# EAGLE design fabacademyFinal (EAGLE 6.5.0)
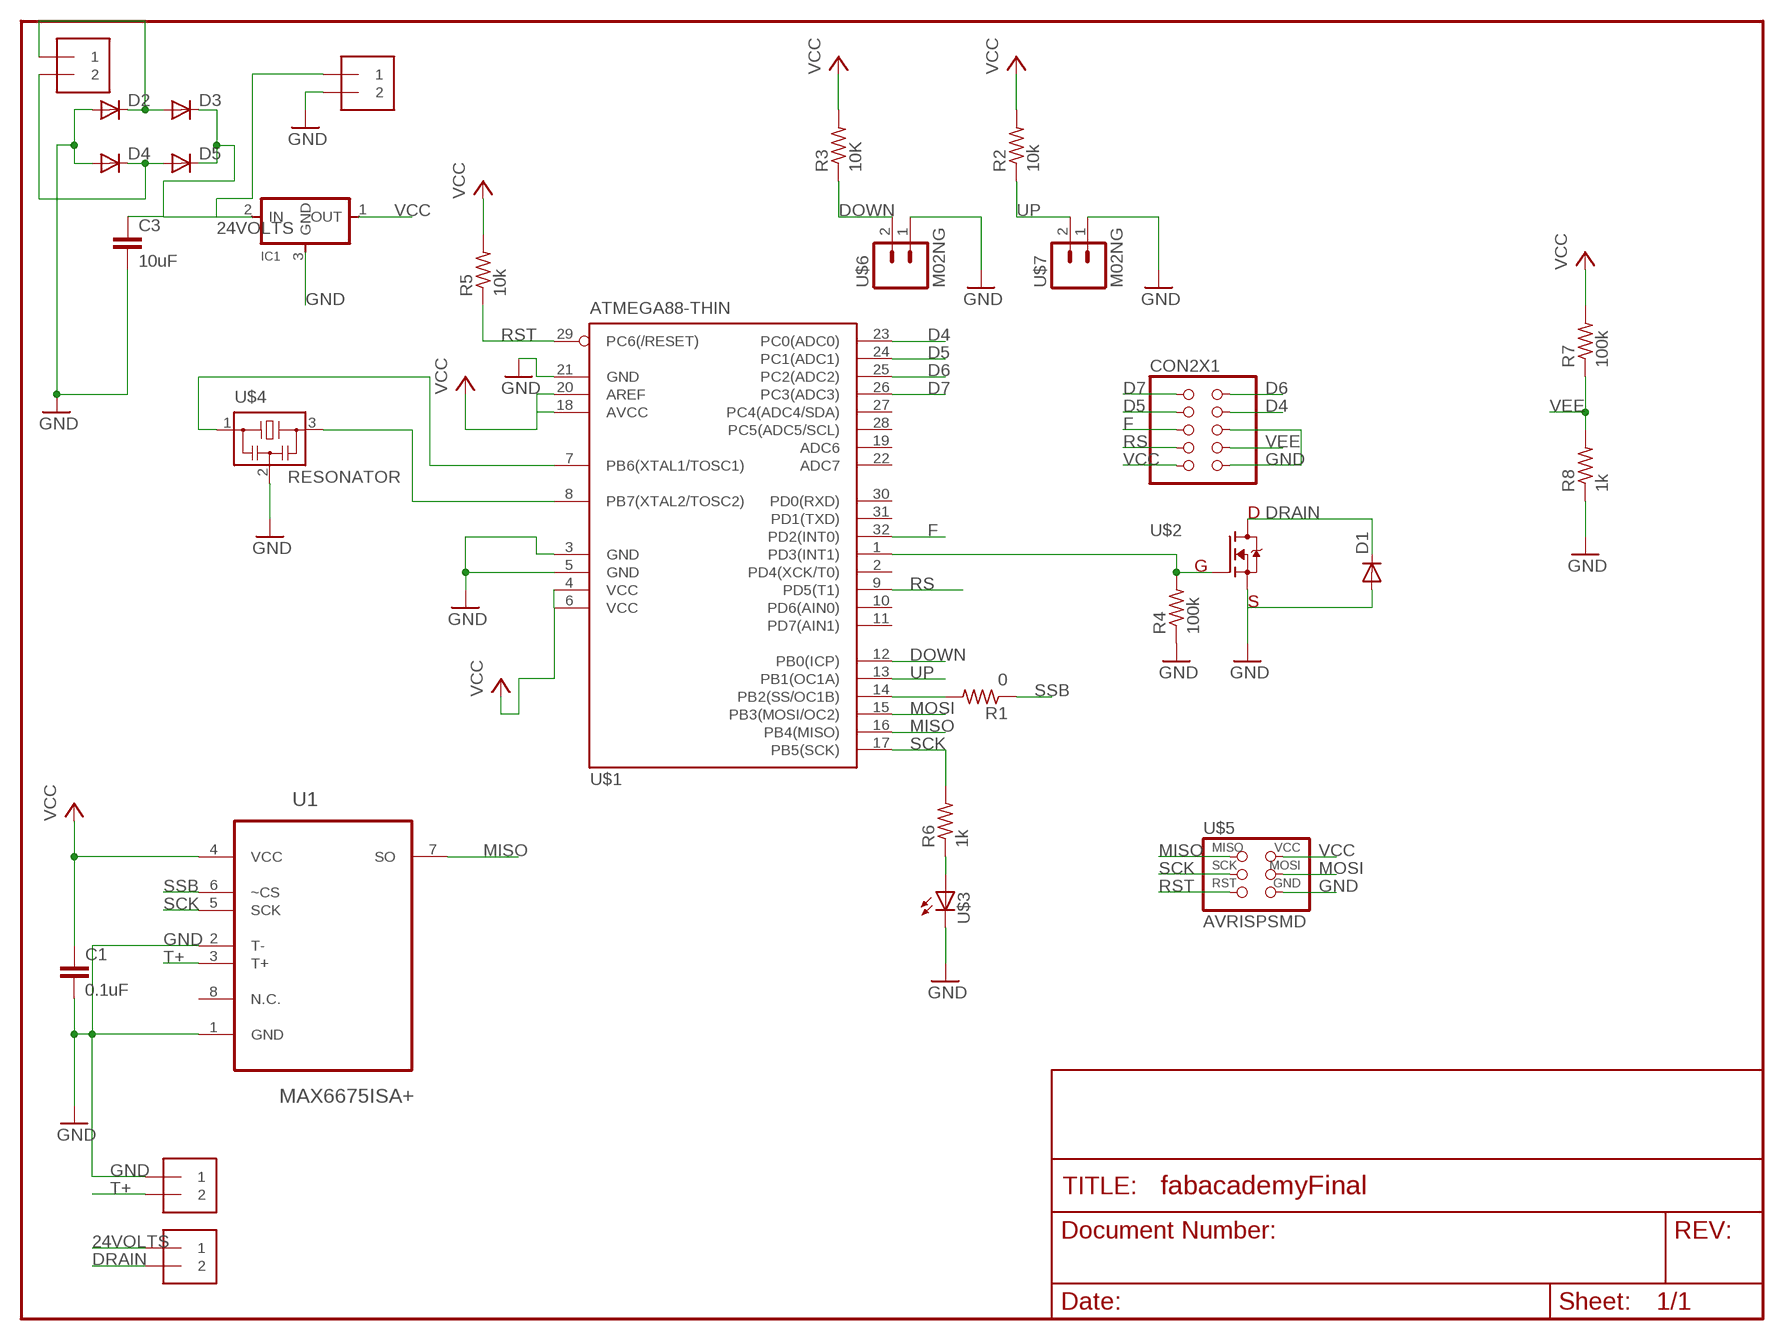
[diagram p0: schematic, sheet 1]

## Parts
C1  0.1uF  CAP1206  [1206]
C3  10uF  CAP1206  [1206]
CON2X1  CONN2X05  [2X05SMD]
D1  DIODESOD123  [SOD123]
D2  DIODESOD123  [SOD123]
D3  DIODESOD123  [SOD123]
D4  DIODESOD123  [SOD123]
D5  DIODESOD123  [SOD123]
IC1  REGULATORSOT23  [SOT23]
J1  1X2-3.5MM  [3.5MMTERM]
J2  1X2-3.5MM  [3.5MMTERM]
J3  1X2-3.5MM  [3.5MMTERM]
J4  1X2-3.5MM  [3.5MMTERM]
R1  0  RESISTOR1206  [1206]
R2  10k  RESISTOR1206  [1206]
R3  10K  RESISTOR1206  [1206]
R4  100k  RESISTOR1206  [1206]
R5  10k  RESISTOR1206  [1206]
R6  1k  RESISTOR1206  [1206]
R7  100k  RESISTOR1206  [1206]
R8  1k  RESISTOR1206  [1206]
U1  MAX6675ISA+  [SOIC127P600X175-8N]
U$1  ATMEGA88-THIN  [TQFP32-08THIN]
U$2  N-MOSFETTO-252  [N-MOSFET]
U$3  LED1206  [1206]
U$4  RESONATOR  [EFOBM]
U$5  AVRISPSMD  [2X03SMD]
U$6  M02NG  [1X02]
U$7  M02NG  [1X02]

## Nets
24VOLTS: C3.1 D3.CATHODE(C) D5.CATHODE(C) IC1.2(IN) J1.1 J2.1
D4: CON2X1.7(DB4) U$1.23(PC0(ADC0))
D5: CON2X1.8(DB5) U$1.24(PC1(ADC1))
D6: CON2X1.9(DB6) U$1.25(PC2(ADC2))
D7: CON2X1.10(DB7) U$1.26(PC3(ADC3))
DOWN: R3.1 U$1.12(PB0(ICP)) U$6.2
DRAIN: D1.CATHODE(C) J2.2 U$2.3(D)
F: CON2X1.6(E) U$1.32(PD2(INT0))
GND: C1.2 C3.2 CON2X1.1(GND) CON2X1.5(R/W) D1.ANODE(A) D2.ANODE(A) D4.ANODE(A) IC1.3(GND) J1.2 J3.1 R4.1 R8.1 U1.1(GND) U1.2(T-) U$1.3(GND) U$1.5(GND) U$1.21(GND) U$2.2(S) U$3.2(C) U$4.2 U$5.6(GND) U$6.1 U$7.1
MISO: U1.7(SO) U$1.16(PB4(MISO)) U$5.1(MISO)
MOSI: U$1.15(PB3(MOSI/OC2)) U$5.4(MOSI)
N$1: D2.CATHODE(C) D3.ANODE(A) J4.1
N$2: D4.CATHODE(C) D5.ANODE(A) J4.2
N$3: R4.2 U$1.1(PD3(INT1)) U$2.1(G)
N$4: U$1.8(PB7(XTAL2/TOSC2)) U$4.3
N$5: U$1.7(PB6(XTAL1/TOSC1)) U$4.1
N$6: R6.1 U$3.1(A)
N$7: R1.2 U$1.14(PB2(SS/OC1B))
RS: CON2X1.4(RS) U$1.9(PD5(T1))
RST: R5.1 U$1.29(PC6(/RESET)) U$5.5(RST)
SCK: R6.2 U1.5(SCK) U$1.17(PB5(SCK)) U$5.3(SCK)
SSB: R1.1 U1.6(~CS)
T+: J3.2 U1.3(T+)
UP: R2.1 U$1.13(PB1(OC1A)) U$7.2
VCC: C1.1 CON2X1.2(VCC) IC1.1(OUT) R2.2 R3.2 R5.2 R7.2 U1.4(VCC) U$1.4(VCC) U$1.6(VCC) U$1.18(AVCC) U$1.20(AREF) U$5.2(VCC)
VEE: CON2X1.3(VEE) R7.1 R8.2
Unconnected: U1.8(N.C.) U$1.2(PD4(XCK/T0)) U$1.10(PD6(AIN0)) U$1.11(PD7(AIN1)) U$1.19(ADC6) U$1.22(ADC7) U$1.27(PC4(ADC4/SDA)) U$1.28(PC5(ADC5/SCL)) U$1.30(PD0(RXD)) U$1.31(PD1(TXD))

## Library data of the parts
C1 C3 = 01_SparkFun:CAP: Capacitor
CON2X1 = 01_ng:CONN2X05
D1-D5 = 01_ng:DIODE: DIODE
IC1 = 01_ng:REGULATOR
J1-J4 = 01_adafruit:1X2: 3.5mm Terminal block
R1-R8 = 01_ng:RESISTOR
U1 = Maxim_By_element14_Batch_1:MAX6675ISA+: Cold-Junction-Compensated K-Thermocoupleto-to-; MPN: MAX6675ISA+; OC_FARNELL: 1379740; OC_NEWARK: 68K4982; PACKAGE: SOIC-8; SUPPLIER: Maxim
U$1 = 01_fab:ATMEGA88-THIN
U$2 = 01_Ali:N-MOSFET
U$3 = 01_ng:LED
U$4 = 01_fab:RESONATOR
U$5 = 01_FAB_Hello:AVRISP
U$6 U$7 = 01_SparkFun:M02NG

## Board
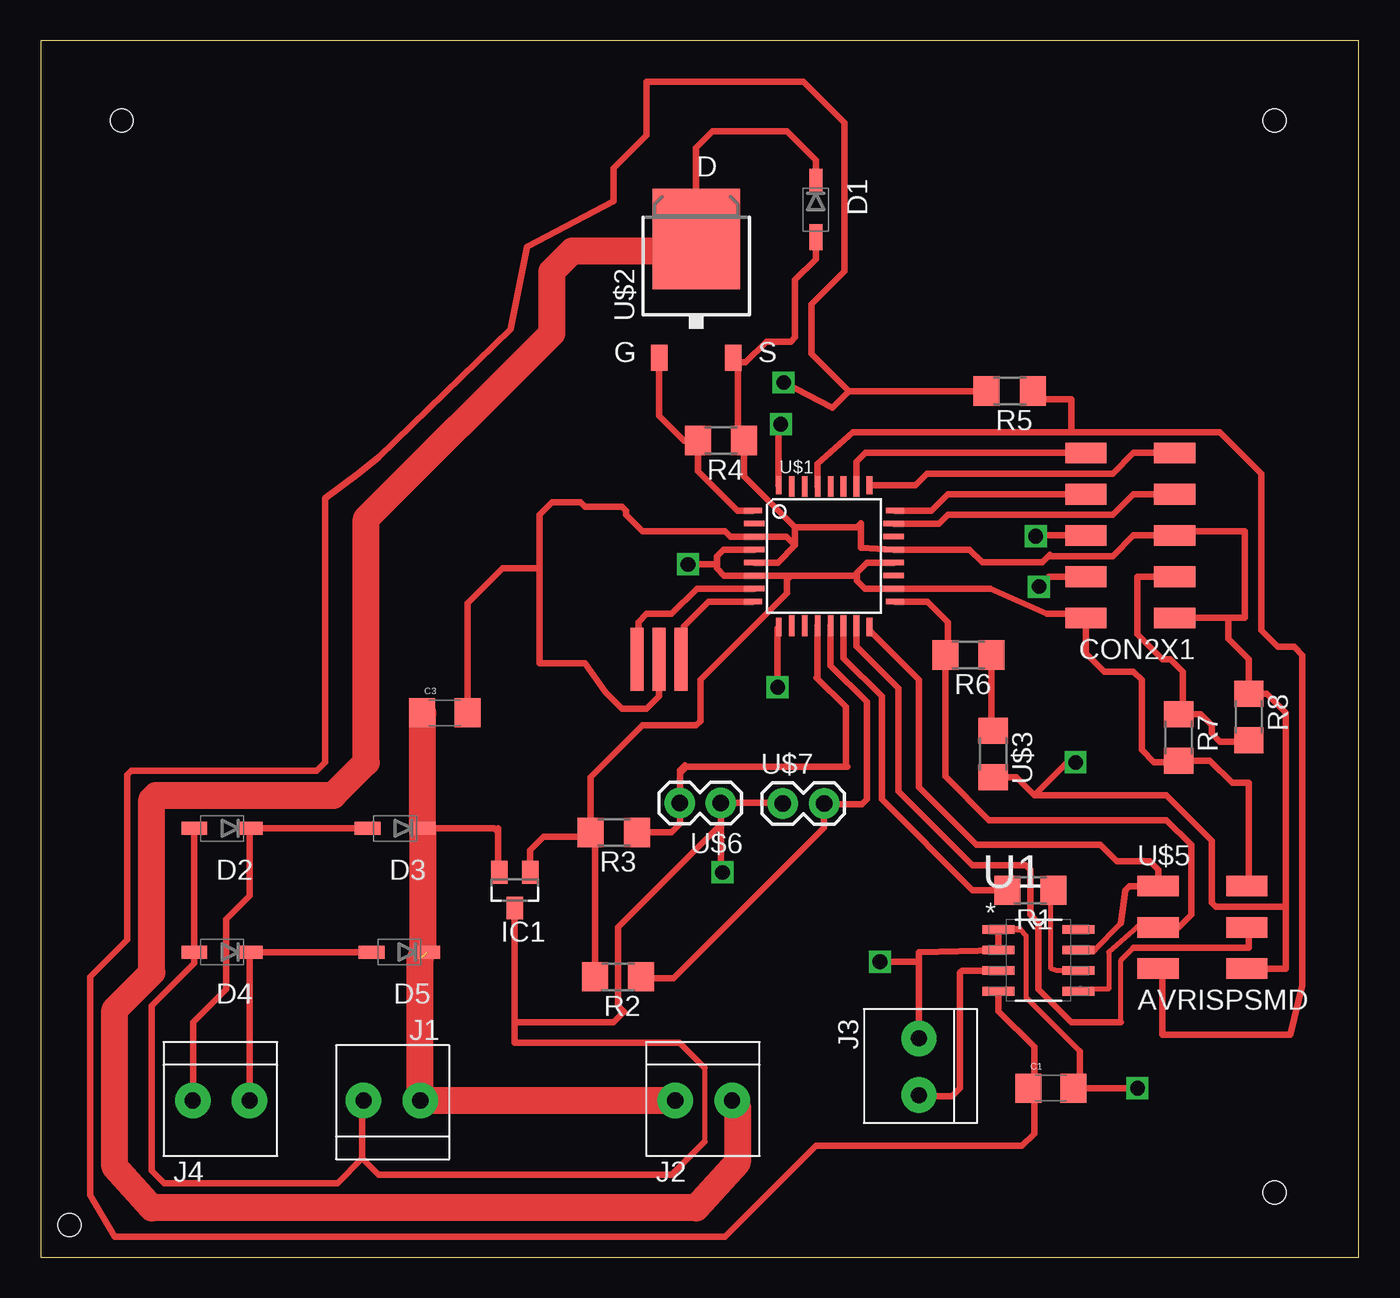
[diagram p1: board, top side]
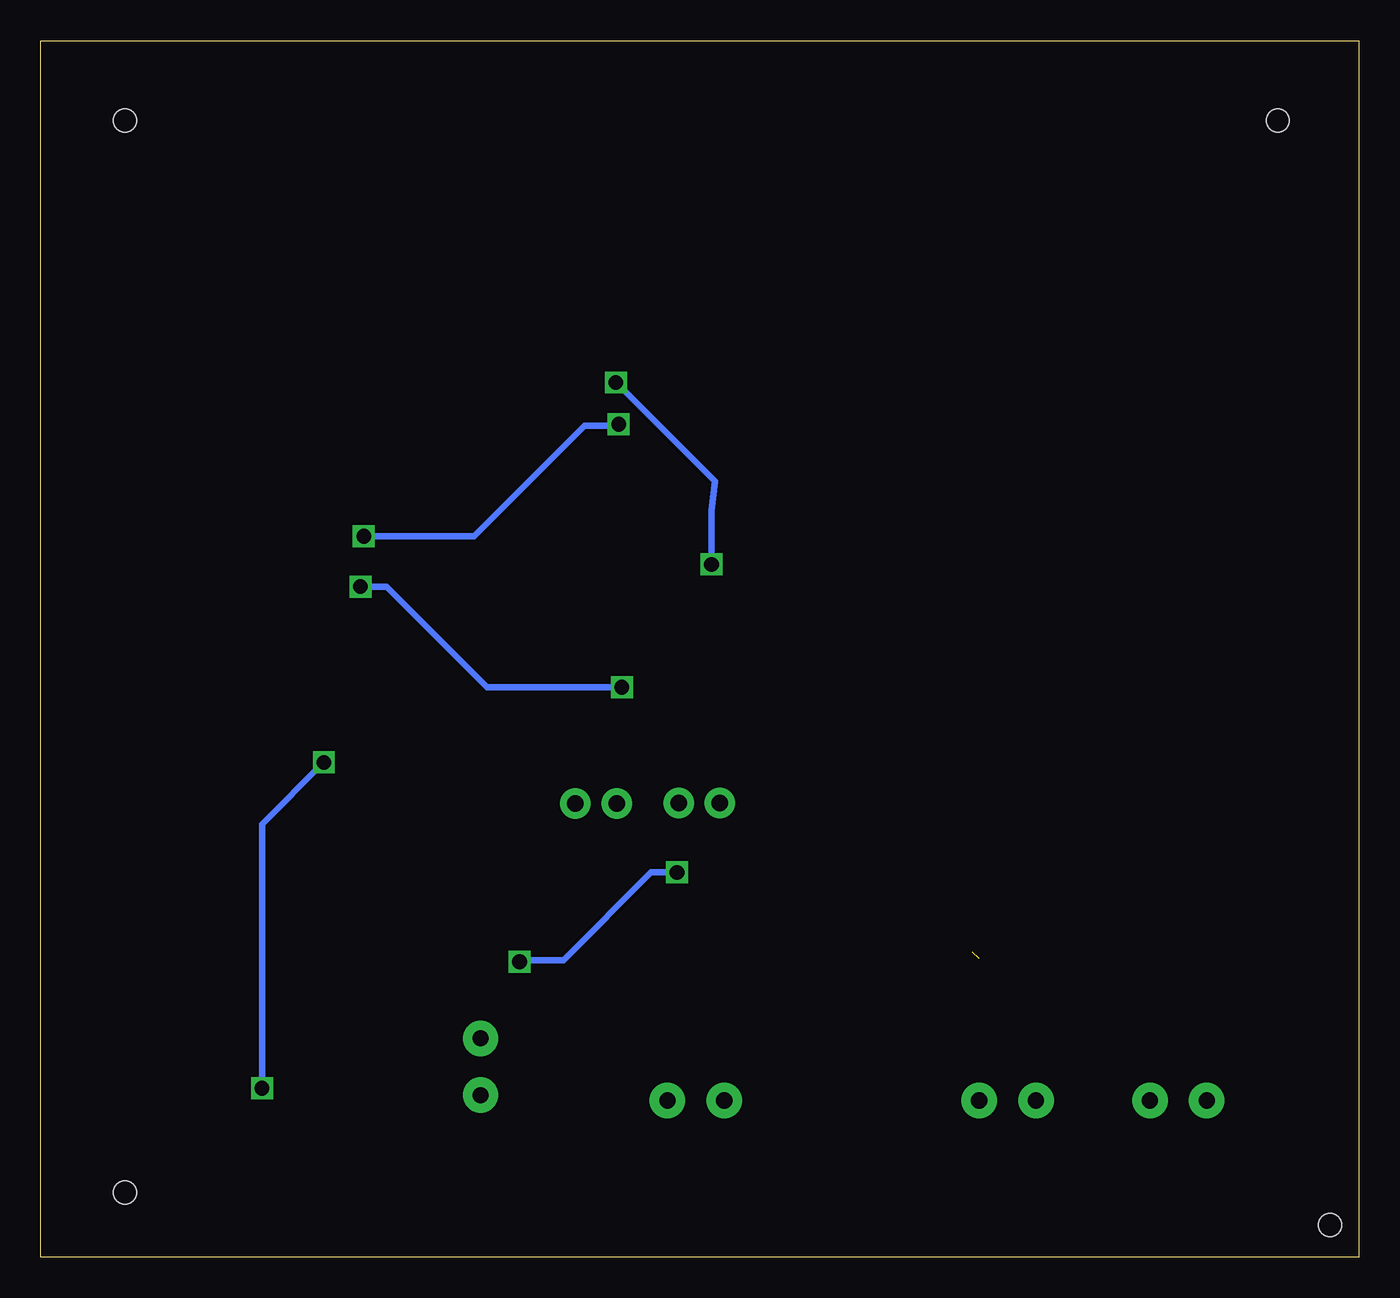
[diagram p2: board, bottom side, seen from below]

Size 81.2 x 74.92 mm. Coordinates in mm from the lower left corner, seen from the top.
Outline: 0,0 81.2,0 81.2,74.92 0,74.92 0,0
Copper layers (1*16): Top 0.035mm / dielectric 1.5mm / Bottom 0.035mm
Design rules "default *": minimum track width 16mil, minimum drill 24mil, track to track 15mil, track to pad 15mil, pad to pad 16mil, via to via 16mil, smd to smd 8mil, copper to edge 40mil, drill to drill 8mil, minimum pad ring 10mil, minimum via ring 8mil, stop-mask expansion 4mil, vias tented up to drill 0mil, thermal gap 10mil
Holes 1.4 mm at 76,70 5,70 76,4 1.78,2

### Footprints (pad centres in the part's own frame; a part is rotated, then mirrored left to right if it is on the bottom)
1206 = smd 1.6 x 1.8: 1 -1.4,0; 2 1.4,0
2X05SMD = smd 2.54 x 1.27: 1 -2.54,3.81; 2 2.92,3.81; 3 -2.54,1.27; 4 2.92,1.27; 5 -2.54,-1.27; 6 2.92,-1.27; 7 -2.54,-3.81; 8 2.92,-3.81; 9 -2.54,-6.35; 10 2.92,-6.35
SOD123 = smd 1.6 x 0.8: ANODE 1.7,0; CATHODE -1.7,0
SOT23 = smd 1 x 1.4: 1 -0.95,-1.1; 2 0.95,-1.1; 3 0,1.1
3.5MMTERM = drill 1 pad 2.184: 1 1.8,0; 2 -1.7,0
1206' = smd 1.6 x 1.803: 1 -1.422,0; 2 1.422,0
SOIC127P600X175-8N = smd 1.981 x 0.533: 1 -2.464,1.905; 2 -2.464,0.635; 3 -2.464,-0.635; 4 -2.464,-1.905; 5 2.464,-1.905; 6 2.464,-0.635; 7 2.464,0.635; 8 2.464,1.905
TQFP32-08THIN = smd 1.118 x 0.356: 1 -4.369,2.8; 8 -4.369,-2.8; 17 4.369,-2.8; 24 4.369,2.8 | smd 1.27 x 0.356: 2 -4.293,2; 3 -4.293,1.2; 4 -4.293,0.4; 5 -4.293,-0.4; 6 -4.293,-1.2; 7 -4.293,-2; 18 4.293,-2; 19 4.293,-1.2; 20 4.293,-0.4; 21 4.293,0.4; 22 4.293,1.2; 23 4.293,2 | smd 0.356 x 1.118: 9 -2.8,-4.369; 16 2.8,-4.369; 25 2.8,4.369; 32 -2.8,4.369 | smd 0.356 x 1.27: 10 -2,-4.293; 14 1.2,-4.293; 15 2,-4.293; 26 2,4.293; 27 1.2,4.293; 31 -2,4.293 | smd 0.35 x 1.27: 11 -1.2,-4.293; 12 -0.4,-4.293; 13 0.4,-4.293; 28 0.4,4.293; 29 -0.4,4.293; 30 -1.2,4.293
N-MOSFET = smd 1 x 1.6: 1 -2.28,-4.8; 2 2.28,-4.8 | smd 5.4 x 6.2: 3 0,2.5
EFOBM = smd 0.8 x 3.9: 1 -1.35,0; 2 0,0; 3 1.35,0
2X03SMD = smd 2.54 x 1.27: 1 -2.54,2.54; 2 2.92,2.54; 3 -2.54,0; 4 2.92,0; 5 -2.54,-2.54; 6 2.92,-2.54
1X02 = drill 1.016 pad 1.88: 1 0,0; 2 2.54,0

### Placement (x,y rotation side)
C1  62.23,10.41 0 top
C3  24.89,33.53 0 top
CON2X1  67.31,43.18 180 top
D1  47.75,64.52 270 top
D2  11.18,26.42 180 top
D3  21.84,26.42 180 top
D4  11.18,18.8 180 top
D5  22.1,18.8 180 top
IC1  29.21,22.61 180 top
J1  21.59,9.65 0 top
J2  40.89,9.65 180 top
J3  54.1,11.68 90 top
J4  11.18,9.65 180 top
R1  0  [1206']  60.96,22.61 180 top
R2  10k  [1206']  35.56,17.27 180 top
R3  10K  [1206']  35.31,26.16 180 top
R4  100k  [1206']  41.91,50.29 180 top
R5  10k  [1206']  59.69,53.34 180 top
R6  1k  [1206']  57.15,37.08 180 top
R7  100k  [1206']  70.1,32 270 top
R8  1k  [1206']  74.42,33.27 270 top
U1  61.47,18.29 0 top
U$1  48.26,43.18 0 top
U$2  40.39,60.2 0 top
U$3  [1206']  58.67,30.99 270 top
U$4  38.1,36.83 0 top
U$5  71.37,20.32 0 top
U$6  41.9,27.98 180 top
U$7  45.72,27.94 0 top

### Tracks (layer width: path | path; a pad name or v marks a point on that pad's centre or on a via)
24VOLTS  (1 unrouted)
  Top 0.406: J1.1 23.39,10.16 23.9,9.65 | 28.19,26.42 28.19,26.16 | 28.19,26.16 28.19,23.77 IC1.2 | 23.54,19.05 D5.CATHODE | 23.54,33.48 C3.1 | D3.CATHODE 27.94,26.42 28.19,26.16
  Top 1.676: 23.39,10.16 23.39,18.39 | J2.1 23.9,9.65 | 23.54,19.05 D3.CATHODE 23.54,33.48
D4
  Top 0.406: U$1.23 55.34,45.18 55.88,45.72 66.04,45.72 67.31,46.99 CON2X1.7
D5
  Top 0.406: U$1.24 54.87,45.98 55.88,46.99 CON2X1.8
D6
  Top 0.406: U$1.25 53.9,47.55 54.61,48.26 66.04,48.26 67.31,49.53 CON2X1.9
D7
  Top 0.406: U$1.26 50.26,48.99 50.8,49.53 CON2X1.10
DOWN
  Top 0.406: R3.1 38.86,26.16 39.4,26.7 39.4,27.94 U$6.2 39.4,28.02 39.4,29.8 | 39.7,30.3 39.4,30 39.4,29.8 | U$1.12 47.86,35.76 47.8,35.7 49.6,33.9 49.6,30.3 49.7,30.2 39.8,30.2 39.4,29.8
DRAIN
  Top 0.406: D1.CATHODE 47.75,67.56 45.97,69.34 41.4,69.34 40.39,68.33 U$2.3 40.35,62.7 39.88,62.23 40.13,61.98 | J2.2 42.93,9.32 | 6.86,28.19 7.11,28.45
  Top 1.676: 42.93,9.32 42.93,5.84 40.39,3.05 6.86,3.05 4.57,5.59 4.57,15.24 6.86,17.53 6.86,28.19 | 7.11,28.45 18.03,28.45 20.07,30.48 20.07,45.47 31.5,56.9 31.5,60.71 32.77,61.98 40.13,61.98
F  (via drill 0.9)
  Top 0.406: CON2X1.6 61.35,44.45 v61.3,44.4 | U$1.32 45.46,51.16 v45.6,51.3
  Bottom 0.406: v61.3,44.4 54.5,44.4 47.7,51.2 46.1,51.2 | 46.1,51.2 45.7,51.2 v45.6,51.3 46,51.3 46.1,51.2
GND  (via drill 0.9)
  Top 0.305: 40.89,11.68 40.89,7.11 | 60.33,20.19 60.71,19.81 60.71,16 64.01,12.7
  Top 0.406: CON2X1.1 73.15,39.37 | 73.15,39.37 74.17,39.37 74.17,44.7 69.85,44.7 CON2X1.5 67.31,44.45 66.04,43.18 62.23,43.18 62.16,43.26 61.7,42.8 58,42.8 57.22,43.58 U$1.21 50.55,43.69 50.55,45.21 50.29,44.96 46.48,44.96 | 73.15,39.37 73.15,38.1 74.42,36.83 R8.1 75.54,34.7 76.71,33.53 76.71,21.59 | 76.71,21.59 76.71,17.78 U$5.6 | U$3.2 60.1,29.57 61.21,28.45 | 61.21,28.45 69.34,28.45 72.14,25.65 72.14,21.84 72.39,21.59 76.71,21.59 | U$4.2 38.1,34.54 37.34,33.78 35.81,33.78 34.8,34.8 33.53,36.58 30.73,36.58 30.73,42.42 | 30.73,42.42 30.73,45.72 31.5,46.48 33.27,46.48 33.53,46.23 35.81,46.23 36.07,45.97 36.07,45.72 37.08,44.7 42.16,44.7 42.49,44.38 U$1.3 45.94,44.38 46.48,43.83 | D2.ANODE D4.ANODE 9.48,18.11 6.86,15.49 6.86,5.33 7.62,4.57 18.29,4.57 19.81,6.1 | 19.81,6.1 19.81,9.57 J1.2 | C3.2 26.29,40.26 28.45,42.42 30.73,42.42 | D1.ANODE 47.75,61.47 46.48,60.2 46.48,56.64 46.23,56.39 44.7,56.39 43.43,55.12 42.95,55.12 | 42.95,55.12 U$2.2 | IC1.3 29.21,14.48 | 29.21,14.48 35.31,14.48 35.94,15.11 35.56,15.49 35.56,20.32 41.9,26.66 U$6.1 | 29.21,14.48 29.21,13.21 39.37,13.21 40.89,11.68 | 40.89,7.11 38.86,5.08 20.83,5.08 19.81,6.1 | 42.95,55.12 42.95,50.68 R4.1 43.33,48.11 46.48,44.96 | 46.48,44.96 46.48,43.83 | J3.1 54.1,18.2 | 54.1,18.2 54.1,18.8 U1.2 U1.1 60.33,20.19 | 61.21,28.45 63.25,30.48 v63.75,30.48 | v67.56,10.41 C1.2 64.01,10.79 64.01,12.7 | 46.48,43.83 45.43,42.78 U$1.5 | U$6.1 45.68,27.98 U$7.1 | U$6.1 41.9,23.9 v42,23.7 | v51.7,18.2 54.1,18.2
  Bottom 0.406: v63.75,30.48 67.56,26.67 v67.56,10.41 | v42,23.7 43.6,23.7 49,18.3 51.6,18.3 v51.7,18.2
MISO
  Top 0.305: 64.9,18.92 66.55,20.57
  Top 0.406: U$1.16 51.06,38.6 54.1,35.56 54.1,28.96 57.66,25.4 65.28,25.4 66.29,24.38 68.33,24.38 68.83,23.88 U$5.1 67.06,22.86 66.8,22.61 66.55,20.57 | U1.7 64.9,18.92
MOSI
  Top 0.305: 66.55,14.48 66.55,18.29 67.31,19.05
  Top 0.406: U$1.15 50.26,37.62 52.83,35.05 52.83,28.7 57.4,24.13 60.71,24.13 60.96,23.88 60.96,21.08 61.47,20.57 61.47,16.51 63.5,14.48 66.55,14.48 | 67.31,19.05 74.42,19.05 74.42,20.19 U$5.4
N$1
  Top 0.406: D3.ANODE D2.CATHODE 12.88,22.27 11.43,20.83 11.43,16.51 9.4,14.48 9.4,9.67 J4.1
N$2
  Top 0.406: D5.ANODE D4.CATHODE J4.2
N$3
  Top 0.406: U$2.1 38.11,51.81 39.62,50.29 R4.2 40.49,48.41 42.92,45.98 U$1.1
N$4
  Top 0.406: U$1.8 41.14,40.38 39.62,38.86 39.62,37 U$4.3
N$5
  Top 0.406: U$1.7 40.42,41.18 38.86,39.62 37.34,39.62 36.83,39.12 36.83,36.91 U$4.1
N$6
  Top 0.406: R6.1 58.57,32.51 U$3.1
N$7
  Top 0.406: U$1.14 49.46,36.9 51.82,34.54 51.82,28.19 57.4,22.61 R1.2
RS  (via drill 0.9)
  Top 0.406: CON2X1.4 62.11,41.91 v61.5,41.3 | v45.4,35.1 45.4,38.75 U$1.9
  Bottom 0.406: v61.5,41.3 59.9,41.3 53.7,35.1 v45.4,35.1
RST
  Top 0.406: U$1.29 47.86,48.88 50.04,50.8 62.74,50.8 63.5,50.8 | 63.5,50.8 72.64,50.8 75.18,48.26 75.18,38.61 76.2,37.59 77.22,37.59 77.72,37.08 77.72,16.76 76.96,13.72 69.09,13.72 69.09,17.53 U$5.5 | 63.5,50.8 63.5,52.83 61.62,52.83 R5.1
SCK
  Top 0.305: 67.56,20.32 65.79,18.8 65.79,16.51 64.06,16.51
  Top 0.406: U$1.17 54.62,40.38 55.88,39.12 55.88,37.24 R6.2 55.73,29.62 58.42,26.92 69.34,26.92 70.87,25.4 70.87,21.08 70.1,20.32 U$5.3 67.56,20.32 | 64.06,16.51 U1.5
SSB
  Top 0.305: U1.6 62.61,17.65 62.23,17.78 62.23,22.5
  Top 0.406: 62.23,22.5 R1.1
T+
  Top 0.406: U1.3 56.77,17.65 56.64,17.53 56.64,10.41 56.13,9.91 54.18,9.91 J3.2
UP
  Top 0.406: U$1.13 48.66,36.44 50.9,34.2 50.9,28.2 50.6,27.9 48.3,27.9 U$7.2 48.26,26.46 39,17.2 37.05,17.2 R2.1
VCC  (via drill 0.9)
  Top 0.406: U$5.2 74.42,22.99 74.42,29.21 73.41,29.21 72.03,30.58 R7.2 70,30.48 68.58,30.48 67.82,31.24 67.82,35.56 67.31,36.07 65.53,36.07 64.39,37.21 CON2X1.2 64.14,39.62 61.98,39.62 58.52,41.18 U$1.18 50.77,41.18 50.29,41.66 50.29,41.91 | U1.4 59,15.16 61.21,12.95 61.21,10.8 C1.1 61.21,10.03 61.21,7.62 60.45,6.86 47.75,6.86 42.16,1.27 4.57,1.27 3.05,3.81 3.05,17.27 5.33,19.56 5.33,29.72 5.59,29.97 17.02,29.97 17.53,30.48 17.53,46.74 19.56,48.26 20.83,49.28 28.96,57.15 29.97,62.23 35.31,65.02 35.31,67.06 37.34,69.09 37.34,72.39 46.99,72.39 49.53,69.85 49.53,60.71 47.5,58.67 47.5,55.63 49.78,53.34 | IC1.1 30.16,25.08 30.99,25.91 33.63,25.91 R3.2 | R2.2 34.14,25.91 R3.2 | U$1.20 50.91,42.78 50.29,42.16 50.29,41.91 | 46.23,41.98 U$1.6 42.09,41.98 41.66,42.42 41.66,42.67 | 46.23,41.98 50.22,41.98 50.29,41.91 | R3.2 33.88,29.57 37.08,32.77 40.39,32.77 40.64,33.02 40.64,35.56 45.97,40.89 45.97,41.73 46.23,41.98 | 41.66,42.67 41.66,43.18 42.06,43.58 U$1.4 | R5.2 49.78,53.34 | 49.78,53.34 48.77,52.32 v45.77,53.87 | v39.88,42.67 41.66,42.67
  Bottom 0.406: v45.77,53.87 39.67,47.77 39.88,45.97 v39.88,42.67
VEE
  Top 0.406: CON2X1.3 67.56,41.91 67.56,38.35 69.09,36.83 69.6,36.83 70.36,36.07 70.36,33.68 R7.1 71.48,33.43 72.14,32.77 72.14,32.26 72.64,31.75 74.32,31.75 R8.2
